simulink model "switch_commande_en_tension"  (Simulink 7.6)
settings: Solver=ode15s  StartTime=0.0  StopTime=0.04  RelTol=1e-3
InitFcn:
  | R1=10e3;
  | R2=R1;
  | R3=R1;
  | clc
StopFcn:
  | close all, clc
  | load signaux.mat
  | plot(x(1,:),x(2,:),x(1,:),x(3,:))
  | grid
  | 
  | title('Switch commandé en tension')
  | xlabel('temps continu')
undefined symbols (not defined in the file or in its folder): sigbuilder_block
libraries: fl_lib x10, nesl_utility x4, elec_lib x4

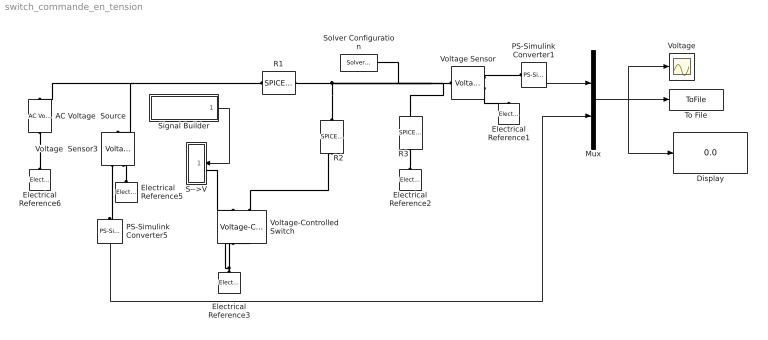
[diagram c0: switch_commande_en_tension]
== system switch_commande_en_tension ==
  AC Voltage  Source : fl_lib/Electrical/Electrical Sources/AC Voltage Source  DialogController=NetworkEngine.DynNeDlgSource  SystemSampleTime=-1  amp=0.1 V  shift=0 rad  omega=100 Hz  i_Log=off  v_Log=off  LocalVarNames=|current|voltage|power  LocalVarDescs=|Current (A)|Voltage (V)|Power (W)  LocalVarLogging=[0 0 0]
  Display : Display
  Electrical Reference{1..3,5..6} (5 alike) : fl_lib/Electrical/Electrical Elements/Electrical Reference  DialogController=NetworkEngine.DynNeDlgSource  SystemSampleTime=-1  i_Log=off  LocalVarNames=|i  LocalVarDescs=|i  LocalVarLogging=[]
  Mux : Mux  Inputs=2
  PS-Simulink Converter1 : nesl_utility/PS-Simulink Converter  DialogController=NetworkEngine.DynNeUtilDlgSource  SystemSampleTime=-1  PhysicalDomain=network_engine_domain  LeftPortType=input  RightPortType=output  SubClassName=ps_output  Unit=1  AffineConversion=off
  PS-Simulink Converter5 : nesl_utility/PS-Simulink Converter  DialogController=NetworkEngine.DynNeUtilDlgSource  SystemSampleTime=-1  PhysicalDomain=network_engine_domain  LeftPortType=input  RightPortType=output  SubClassName=ps_output  Unit=1  AffineConversion=off
  R1 : elec_lib/Additional Components/SPICE-Compatible Components/Passive Devices/SPICE Resistor  DialogController=NetworkEngine.DynNeDlgSource  SystemSampleTime=-1  SCALE=1  R_param=1  R=R1 Ohm  RSH=0 Ohm  LENGTH=1e-06 m  WIDTH=1e-06 m  NARROW=0 m  T_param=1  TC1=0 1/K  TC2=0 1/K^2  TOFFSET=0 K  TFIXED=300.15 K  TMEAS=300.15 K  LocalVarLogging=[]
  R2 : elec_lib/Additional Components/SPICE-Compatible Components/Passive Devices/SPICE Resistor  DialogController=NetworkEngine.DynNeDlgSource  SystemSampleTime=-1  SCALE=1  R_param=1  R=R2 Ohm  RSH=0 Ohm  LENGTH=1e-06 m  WIDTH=1e-06 m  NARROW=0 m  T_param=1  TC1=0 1/K  TC2=0 1/K^2  TOFFSET=0 K  TFIXED=300.15 K  TMEAS=300.15 K  LocalVarLogging=[]
  R3 : elec_lib/Additional Components/SPICE-Compatible Components/Passive Devices/SPICE Resistor  DialogController=NetworkEngine.DynNeDlgSource  SystemSampleTime=-1  SCALE=1  R_param=1  R=R3 Ohm  RSH=0 Ohm  LENGTH=1e-06 m  WIDTH=1e-06 m  NARROW=0 m  T_param=1  TC1=0 1/K  TC2=0 1/K^2  TOFFSET=0 K  TFIXED=300.15 K  TMEAS=300.15 K  LocalVarLogging=[]
  S-->V : Subsystem
  Signal Builder : Subsystem  Tag=STV Subsys  LoadFcn=sigbuilder_block('load');  StartFcn=sigbuilder_block('start');  StopFcn=sigbuilder_block('stop');  ClipboardFcn=sigbuilder_block('clipboard');
  Solver Configuration : nesl_utility/Solver Configuration  DialogController=NetworkEngine.DynNeUtilDlgSource  SystemSampleTime=-1  PhysicalDomain=network_engine_domain  LeftPortType=input  RightPortType=generic  SubClassName=solver  Accelerate=off  Profile=off  ResidualTolerance=1e-9  MaxNonlinIter=12  MaxModeIter=2  DoFixedCost=off  UseLocalSampling=off  DoDC=off  LinearAlgebra=Sparse  LocalSolverSampleTime=.001  LocalSolverChoice=NE_BACKWARD_EULER_ADVANCER  UseLocalSolver=off
  To File : ToFile  Filename=signaux  MatrixName=x
  Voltage : Scope
  Voltage  Sensor3 : fl_lib/Electrical/Electrical Sensors/Voltage Sensor  DialogController=NetworkEngine.DynNeDlgSource  SystemSampleTime=-1  i1_Log=off  v1_Log=off  LocalVarNames=|i1|v1  LocalVarDescs=|i1|v1  LocalVarLogging=[0 0]
  Voltage Sensor : fl_lib/Electrical/Electrical Sensors/Voltage Sensor  DialogController=NetworkEngine.DynNeDlgSource  SystemSampleTime=-1  i1_Log=off  v1_Log=off  LocalVarNames=|i1|v1  LocalVarDescs=|i1|v1  LocalVarLogging=[0 0]
  Voltage-Controlled Switch : elec_lib/Additional Components/SPICE-Compatible Components/Passive Devices/Voltage-Controlled Switch  DialogController=NetworkEngine.DynNeDlgSource  SystemSampleTime=-1  VT=0.5 V  VH=0 V  RON=0.001 Ohm  ROFF=1e+12 Ohm  IC_state=-1  LocalVarLogging=[]
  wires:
  PS-Simulink Converter1/1 -> Mux/1
  Mux/1 -> To File/1, Voltage/1, Display/1
  PS-Simulink Converter5/1 -> Mux/2
  Signal Builder/1(Signal 2) -> S-->V/1(s)
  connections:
  Voltage Sensor/RConn2 -- Electrical Reference1/LConn1
  Voltage Sensor/RConn1 -- PS-Simulink Converter1/LConn1
  R1/LConn1 -- AC Voltage  Source/LConn1 -- Voltage  Sensor3/LConn1
  R2/LConn1 -- Voltage Sensor/LConn1 -- R3/LConn1 -- Solver Configuration/RConn1 -- R1/RConn1
  R3/RConn1 -- Electrical Reference2/LConn1
  Voltage-Controlled Switch/LConn2 -- R2/RConn1
  Electrical Reference3/LConn1 -- Voltage-Controlled Switch/RConn1 -- Voltage-Controlled Switch/RConn2
  Voltage  Sensor3/RConn1 -- PS-Simulink Converter5/LConn1
  Electrical Reference5/LConn1 -- Voltage  Sensor3/RConn2
  Electrical Reference6/LConn1 -- AC Voltage  Source/RConn1
  S-->V/LConn1 -- Voltage-Controlled Switch/LConn1

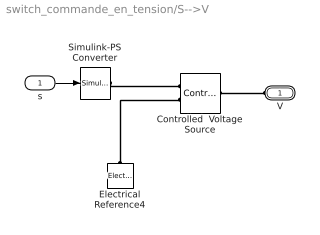
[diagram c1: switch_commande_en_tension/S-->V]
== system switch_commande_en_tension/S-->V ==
  s : Inport
  Controlled  Voltage Source : fl_lib/Electrical/Electrical Sources/Controlled Voltage Source  DialogController=NetworkEngine.DynNeDlgSource  SystemSampleTime=-1  i_Log=off  v_Log=off  LocalVarNames=|i|v  LocalVarDescs=|i|v  LocalVarLogging=[0 0]
  Electrical Reference4 : fl_lib/Electrical/Electrical Elements/Electrical Reference  DialogController=NetworkEngine.DynNeDlgSource  SystemSampleTime=-1  i_Log=off  LocalVarNames=|i  LocalVarDescs=|i  LocalVarLogging=[]
  Simulink-PS Converter : nesl_utility/Simulink-PS Converter  DialogController=NetworkEngine.DynNeUtilDlgSource  SystemSampleTime=-1  PhysicalDomain=network_engine_domain  LeftPortType=input  RightPortType=output  SubClassName=ps_input  Unit=1  AffineConversion=off  InputFilterTimeConstant=.001  UdotUserProvided=0
  V : PMIOPort  Port=1  Side=Left
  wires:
  s/1 -> Simulink-PS Converter/1
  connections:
  Simulink-PS Converter/RConn1 -- Controlled  Voltage Source/RConn1
  Electrical Reference4/LConn1 -- Controlled  Voltage Source/RConn2
  V/RConn1 -- Controlled  Voltage Source/LConn1

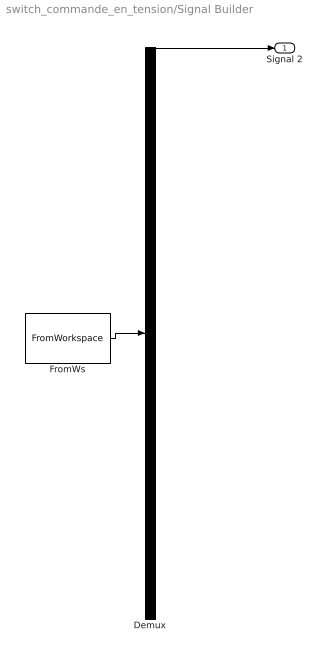
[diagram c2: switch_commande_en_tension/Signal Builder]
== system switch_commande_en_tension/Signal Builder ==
  Demux : Demux  Tag=STV Demux  Outputs=1
  FromWs : FromWorkspace  Tag=STV FromWs  VariableName=tuvar  SampleTime=0  SigBuilderData=DataTag0  VnvData=DataTag1
  Signal 2 : Outport  Tag=STV Outport
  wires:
  FromWs/1 -> Demux/1
  Demux/1 -> Signal 2/1
